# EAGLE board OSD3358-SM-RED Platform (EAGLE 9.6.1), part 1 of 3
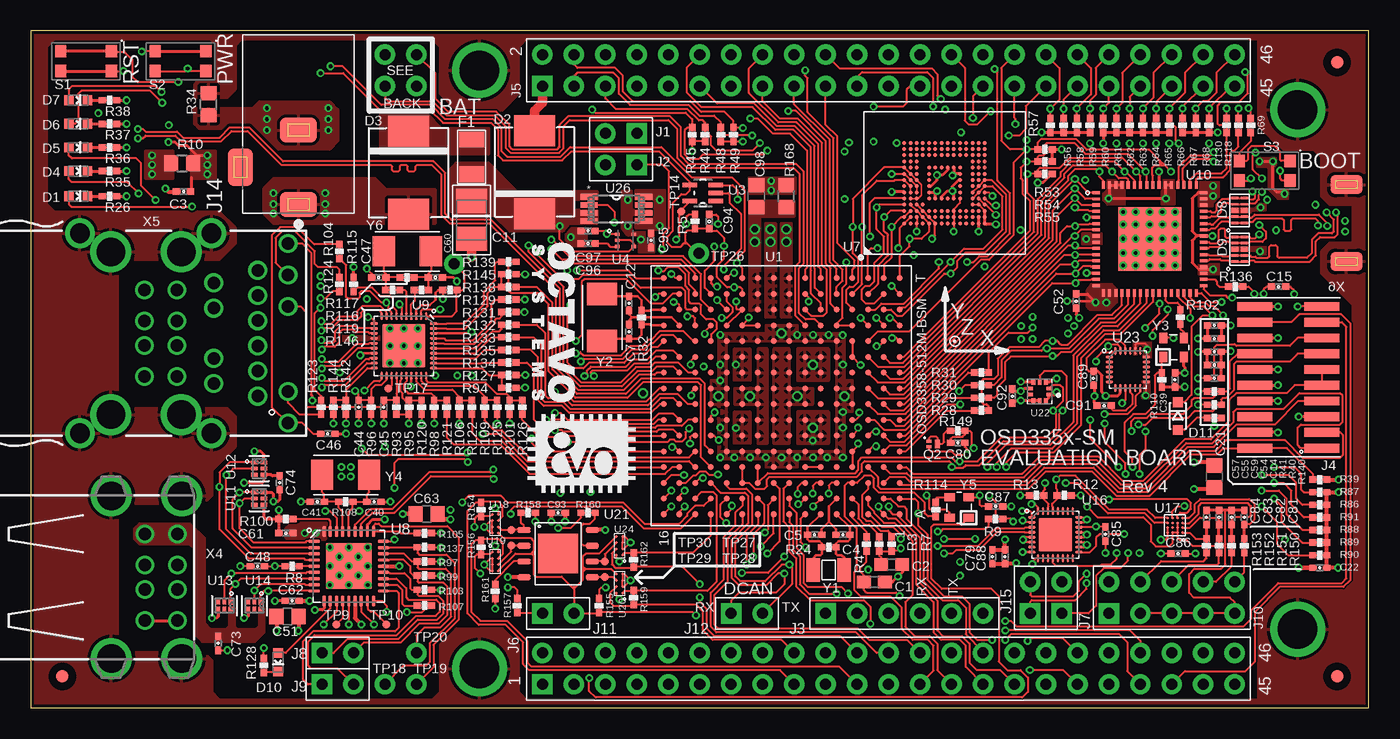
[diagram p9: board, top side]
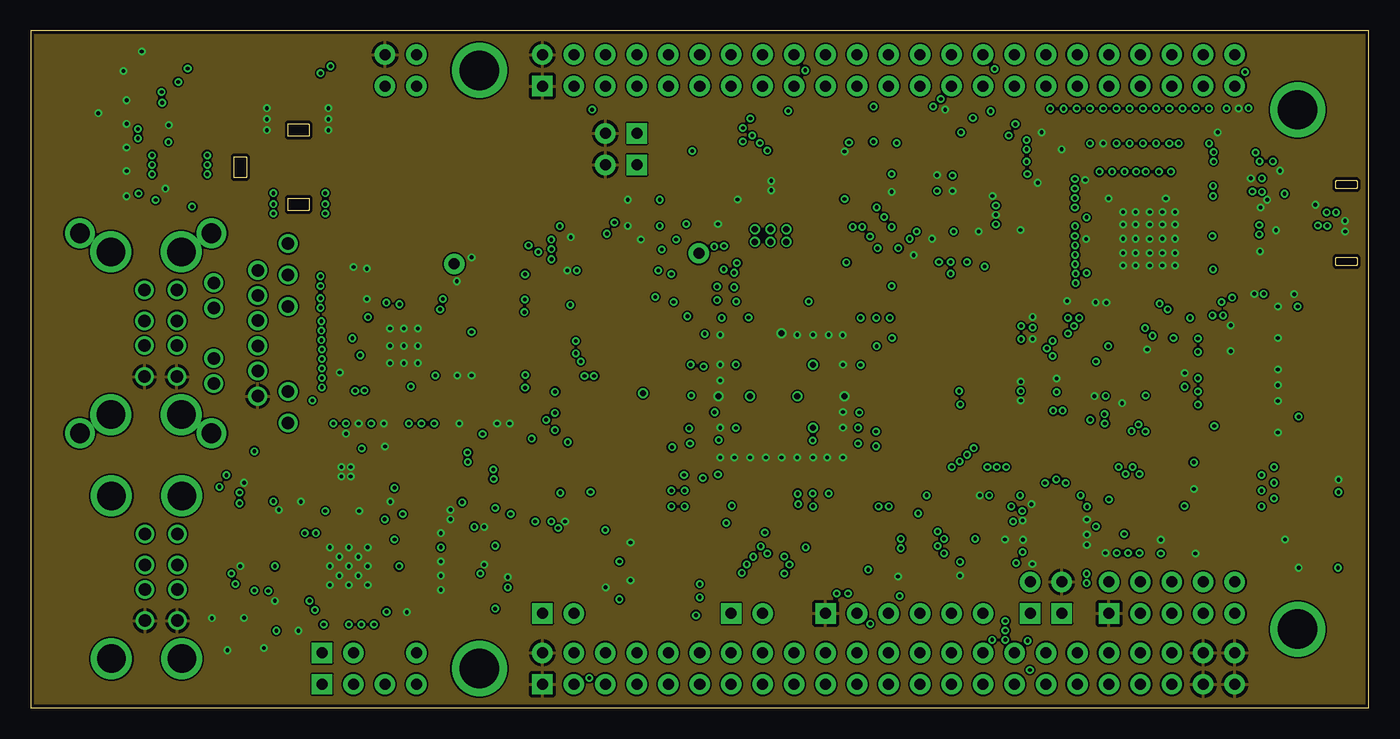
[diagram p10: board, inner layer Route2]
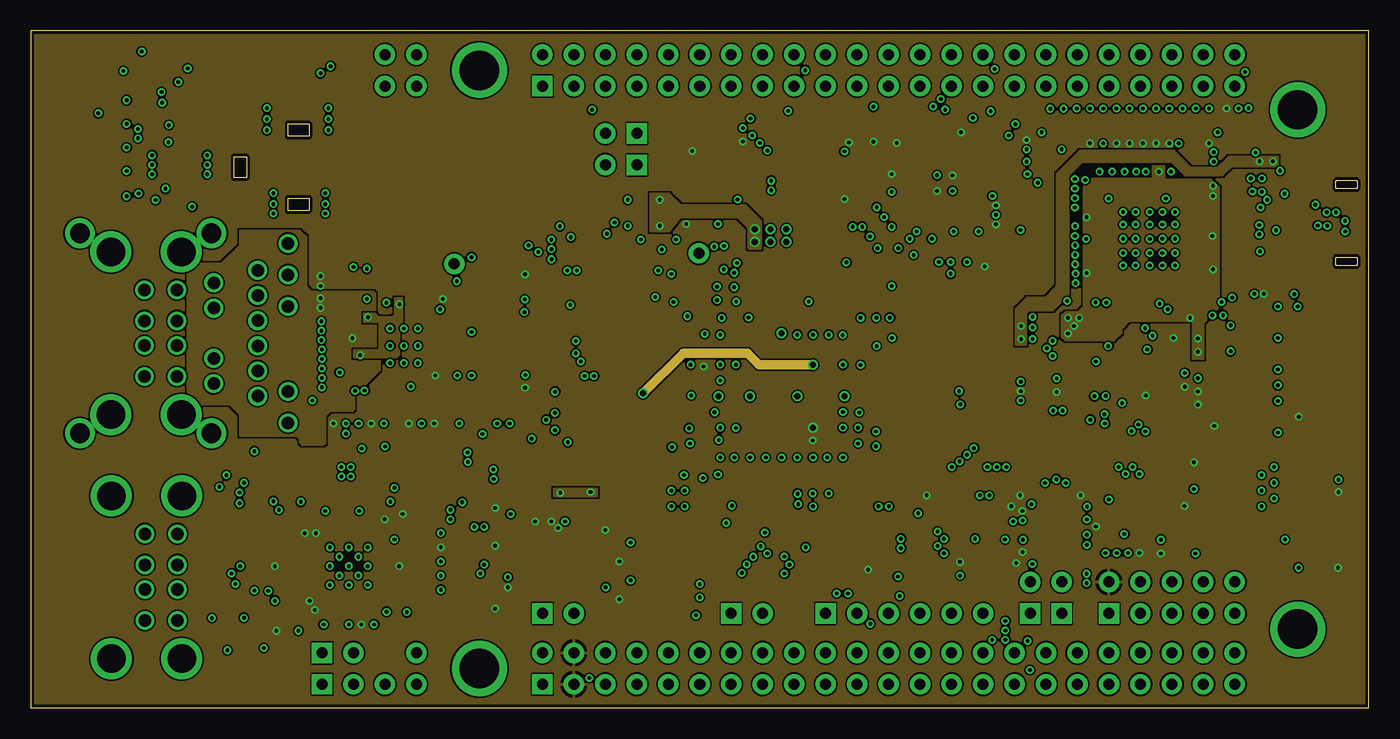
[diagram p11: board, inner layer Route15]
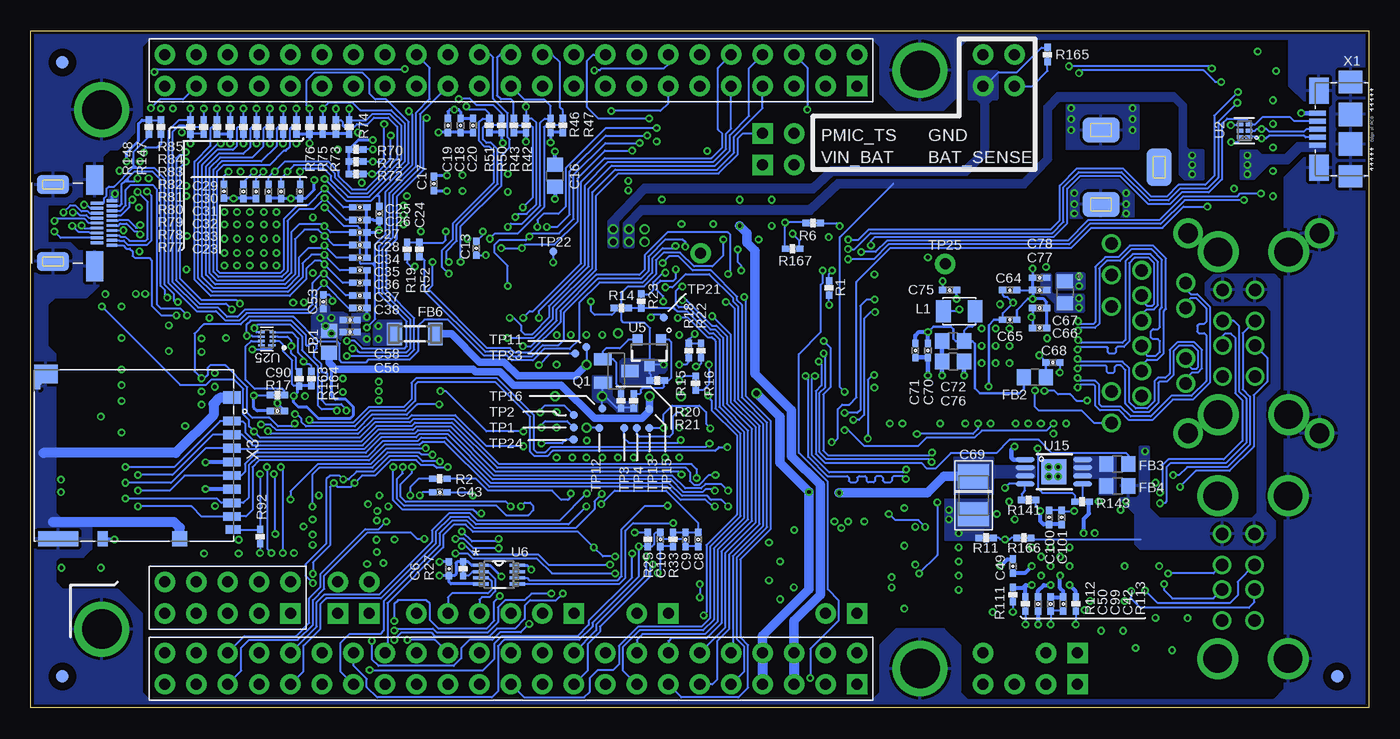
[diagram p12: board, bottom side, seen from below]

Size 107.95 x 54.61 mm. Coordinates in mm from the lower left corner, seen from the top.
Outline: 0,0 107.95,0 107.95,54.61 0,54.61 0,0
Copper layers (1*2*15*16): Top 0.035mm / dielectric 0.23mm / Route2 0.035mm / dielectric 0.93mm / Route15 0.035mm / dielectric 0.23mm / Bottom 0.035mm
Design rules "MF_Standard_4_Layer *": minimum track width 5mil, minimum drill 12mil, track to track 5mil, track to pad 5mil, pad to pad 5mil, via to via 5mil, smd to smd 0mil, copper to edge 10mil, drill to drill 10mil, minimum pad ring 6mil, minimum via ring 6mil, stop-mask expansion 2mil, vias tented up to drill 25mil, thermal gap 10mil
Net classes: 0 default: width 0.127 mm, drill 0.254 mm; 1 ground: width 0.152 mm, drill 0.254 mm, clearance 0.152 mm

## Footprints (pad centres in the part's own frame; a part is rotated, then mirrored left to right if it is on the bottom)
C0603 = smd 1.1 x 1: 1 -0.85,0; 2 0.85,0
C0402 = smd 0.61 x 0.508: 1 -0.559,0; 2 0.559,0
B/3528-21R = smd 1.95 x 2.5: + 1.525,0; - -1.525,0
C0805 = smd 1.143 x 1.27: 1 -0.889,0; 2 0.889,0
0603 = smd 0.787 x 0.787: 1 -0.749,0; 2 0.749,0
SMC = smd 2.5 x 3.3: A 3.35,0; C -3.35,0
10-USON(2.5X1) = smd 0.2 x 0.565: 1 -1,0.385; 2 -0.5,0.385; 4 0.5,0.385; 5 1,0.385; 6 1,-0.385; 7 0.5,-0.385; 9 -0.5,-0.385; 10 -1,-0.385 | smd 0.4 x 0.565: 3 0,0.385; 8 0,-0.385
SOD323(NXP)REFLOW = smd 0.8 x 0.8: A 1.125,0; C -1.125,0
F1206W = smd 1.27 x 2.032: 1 -1.397,0; 2 1.397,0
SM-1206 = smd 1.2 x 1.8: 1 -1.65,0; 2 1.65,0
FIDUCIAL_40MIL = smd 1.016 x 1.016: P$1 0,0
H2-2.54 = drill 0.889 pad 1.651 square: 1 0,1.27 | drill 0.889 pad 1.651: 2 0,-1.27
H6-2.54 = drill 0.889 pad 1.651 square: 1 0,6.35 | drill 0.889 pad 1.651: 2 0,3.81; 3 0,1.27; 4 0,-1.27; 5 0,-3.81; 6 0,-6.35
2ROWS_10PINS_1.27MM_PITCH_ROW_2.54MM_PITCH_PIN6_KEYED = smd 2.794 x 0.711: 1 -2.705,5.715; 2 2.705,5.715; 3 -2.705,4.445; 4 2.705,4.445; 5 -2.705,3.175; 6 2.705,3.175; 7 -2.705,1.905; 8 2.705,1.905; 9 -2.705,0.635; 10 2.705,0.635; 11 -2.705,-0.635; 12 2.705,-0.635; 13 -2.705,-1.905; 14 2.705,-1.905; 15 -2.705,-3.175; 16 2.705,-3.175; 17 -2.705,-4.445; 18 2.705,-4.445; 19 -2.705,-5.715; 20 2.705,-5.715
H2X23-2.54 = drill 0.889 pad 1.651 square: 1 -1.27,27.94 | drill 0.889 pad 1.651: 2 1.27,27.94; 3 -1.27,25.4; 4 1.27,25.4; 5 -1.27,22.86; 6 1.27,22.86; 7 -1.27,20.32; 8 1.27,20.32; 9 -1.27,17.78; 10 1.27,17.78; 11 -1.27,15.24; 12 1.27,15.24; 13 -1.27,12.7; 14 1.27,12.7; 15 -1.27,10.16; 16 1.27,10.16; 17 -1.27,7.62; 18 1.27,7.62; 19 -1.27,5.08; 20 1.27,5.08; 21 -1.27,2.54; 22 1.27,2.54; 23 -1.27,0; 24 1.27,0; 25 -1.27,-2.54; 26 1.27,-2.54; 27 -1.27,-5.08; 28 1.27,-5.08; 29 -1.27,-7.62; 30 1.27,-7.62; 31 -1.27,-10.16; 32 1.27,-10.16; 33 -1.27,-12.7; 34 1.27,-12.7; 35 -1.27,-15.24; 36 1.27,-15.24; 37 -1.27,-17.78; 38 1.27,-17.78; 39 -1.27,-20.32; 40 1.27,-20.32; 41 -1.27,-22.86; 42 1.27,-22.86; 43 -1.27,-25.4; 44 1.27,-25.4; 45 -1.27,-27.94; 46 1.27,-27.94
H2X5-2.54 = drill 0.889 pad 1.651 square: 1 -1.27,5.08 | drill 0.889 pad 1.651: 2 1.27,5.08; 3 -1.27,2.54; 4 1.27,2.54; 5 -1.27,0; 6 1.27,0; 7 -1.27,-2.54; 8 1.27,-2.54; 9 -1.27,-5.08; 10 1.27,-5.08
CUI_PJ-102BH-DIM-SMT-PAD = smd 2 x 3: 1 -6.5,0; 2 -0.5,0 | smd 2 x 3 bottom: 1_B -6.5,0; 2_B -0.5,0 | smd 3 x 2: 3 -3.5,4.7 | smd 3 x 2 bottom: 3_B -3.5,4.7
CVH252009 = smd 1.2 x 1.75: P$1 -1.275,0; P$2 1.275,0
MOUNTING_HOLE = drill 3.175 pad 4.445: P$1 0,0
SOT23-BEC = smd 1 x 1.4: B -0.95,-1.1; C 0,1.1; E 0.95,-1.1
X1-DFN1006-3 = smd 0.4 x 0.25: B -0.35,0.225; E -0.35,-0.225 | smd 0.4 x 0.7: C 0.35,0
R0402 = smd 0.61 x 0.508: 1 -0.559,0; 2 0.559,0
R0805 = smd 1.143 x 1.27: 1 -0.889,0; 2 0.889,0
SW4SMD_63X161LS = smd 0.9 x 1: 1 2.05,0.8; 2 2.05,-0.8; 3 -2.05,0.8; 4 -2.05,-0.8
TP_B0,65 = smd 0.635 x 0.635: TP 0,0
TESTPAD/W_HOLE_1X1 = drill 0.889 pad 1.651: P$1 0,0
OSD335X-BGA-256 = smd 0.5 x 0.5: A1 -9.525,-9.525; A2 -9.525,-8.255; A3 -9.525,-6.985; A4 -9.525,-5.715; A5 -9.525,-4.445; A6 -9.525,-3.175; A7 -9.525,-1.905; A8 -9.525,-0.635; A9 -9.525,0.635; A10 -9.525,1.905; A11 -9.525,3.175; A12 -9.525,4.445; A13 -9.525,5.715; A14 -9.525,6.985; A15 -9.525,8.255; A16 -9.525,9.525; B1 -8.255,-9.525; B2 -8.255,-8.255; B3 -8.255,-6.985; B4 -8.255,-5.715; B5 -8.255,-4.445; B6 -8.255,-3.175; B7 -8.255,-1.905; B8 -8.255,-0.635; B9 -8.255,0.635; B10 -8.255,1.905; B11 -8.255,3.175; B12 -8.255,4.445; B13 -8.255,5.715; B14 -8.255,6.985; B15 -8.255,8.255; B16 -8.255,9.525; C1 -6.985,-9.525; C2 -6.985,-8.255; C3 -6.985,-6.985; C4 -6.985,-5.715; C5 -6.985,-4.445; C6 -6.985,-3.175; C7 -6.985,-1.905; C8 -6.985,-0.635; C9 -6.985,0.635; C10 -6.985,1.905; C11 -6.985,3.175; C12 -6.985,4.445; C13 -6.985,5.715; C14 -6.985,6.985; C15 -6.985,8.255; C16 -6.985,9.525; D1 -5.715,-9.525; D2 -5.715,-8.255; D3 -5.715,-6.985; D4 -5.715,-5.715; D5 -5.715,-4.445; D6 -5.715,-3.175; D7 -5.715,-1.905; D8 -5.715,-0.635; D9 -5.715,0.635; D10 -5.715,1.905; D11 -5.715,3.175; D12 -5.715,4.445; D13 -5.715,5.715; D14 -5.715,6.985; D15 -5.715,8.255; D16 -5.715,9.525; E1 -4.445,-9.525; E2 -4.445,-8.255; E3 -4.445,-6.985; E4 -4.445,-5.715; E5 -4.445,-4.445; E6 -4.445,-3.175; E7 -4.445,-1.905; E8 -4.445,-0.635; E9 -4.445,0.635; E10 -4.445,1.905; E11 -4.445,3.175; E12 -4.445,4.445; E13 -4.445,5.715; E14 -4.445,6.985; E15 -4.445,8.255; E16 -4.445,9.525; F1 -3.175,-9.525; F2 -3.175,-8.255; F3 -3.175,-6.985; F4 -3.175,-5.715; F5 -3.175,-4.445; F6 -3.175,-3.175; F7 -3.175,-1.905; F8 -3.175,-0.635; F9 -3.175,0.635; F10 -3.175,1.905; F11 -3.175,3.175; F12 -3.175,4.445; F13 -3.175,5.715; F14 -3.175,6.985; F15 -3.175,8.255; F16 -3.175,9.525; G1 -1.905,-9.525; G2 -1.905,-8.255; G3 -1.905,-6.985; G4 -1.905,-5.715; G5 -1.905,-4.445; G6 -1.905,-3.175; G7 -1.905,-1.905; G8 -1.905,-0.635; G9 -1.905,0.635; G10 -1.905,1.905; G11 -1.905,3.175; G12 -1.905,4.445; G13 -1.905,5.715; G14 -1.905,6.985; G15 -1.905,8.255; G16 -1.905,9.525; H1 -0.635,-9.525; H2 -0.635,-8.255; H3 -0.635,-6.985; H4 -0.635,-5.715; H5 -0.635,-4.445; H6 -0.635,-3.175; H7 -0.635,-1.905; H8 -0.635,-0.635; H9 -0.635,0.635; H10 -0.635,1.905; H11 -0.635,3.175; H12 -0.635,4.445; H13 -0.635,5.715; H14 -0.635,6.985; H15 -0.635,8.255; H16 -0.635,9.525; J1 0.635,-9.525; J2 0.635,-8.255; J3 0.635,-6.985; J4 0.635,-5.715; J5 0.635,-4.445; J6 0.635,-3.175; J7 0.635,-1.905; J8 0.635,-0.635; J9 0.635,0.635; J10 0.635,1.905; J11 0.635,3.175; J12 0.635,4.445; J13 0.635,5.715; J14 0.635,6.985; J15 0.635,8.255; J16 0.635,9.525; K1 1.905,-9.525; K2 1.905,-8.255; K3 1.905,-6.985; K4 1.905,-5.715; K5 1.905,-4.445; K6 1.905,-3.175; K7 1.905,-1.905; K8 1.905,-0.635; K9 1.905,0.635; K10 1.905,1.905; K11 1.905,3.175; K12 1.905,4.445; K13 1.905,5.715; K14 1.905,6.985; K15 1.905,8.255; K16 1.905,9.525; L1 3.175,-9.525; L2 3.175,-8.255; L3 3.175,-6.985; L4 3.175,-5.715; L5 3.175,-4.445; L6 3.175,-3.175; L7 3.175,-1.905; L8 3.175,-0.635; L9 3.175,0.635; L10 3.175,1.905; L11 3.175,3.175; L12 3.175,4.445; L13 3.175,5.715; L14 3.175,6.985; L15 3.175,8.255; L16 3.175,9.525; M1 4.445,-9.525; M2 4.445,-8.255; M3 4.445,-6.985; M4 4.445,-5.715; M5 4.445,-4.445; M6 4.445,-3.175; M7 4.445,-1.905; M8 4.445,-0.635; M9 4.445,0.635; M10 4.445,1.905; M11 4.445,3.175; M12 4.445,4.445; M13 4.445,5.715; M14 4.445,6.985; M15 4.445,8.255; M16 4.445,9.525; N1 5.715,-9.525; N2 5.715,-8.255; N3 5.715,-6.985; N4 5.715,-5.715; N5 5.715,-4.445; N6 5.715,-3.175; N7 5.715,-1.905; N8 5.715,-0.635; N9 5.715,0.635; N10 5.715,1.905; N11 5.715,3.175; N12 5.715,4.445; N13 5.715,5.715; N14 5.715,6.985; N15 5.715,8.255; N16 5.715,9.525; P1 6.985,-9.525; P2 6.985,-8.255; P3 6.985,-6.985; P4 6.985,-5.715; P5 6.985,-4.445; P6 6.985,-3.175; P7 6.985,-1.905; P8 6.985,-0.635; P9 6.985,0.635; P10 6.985,1.905; P11 6.985,3.175; P12 6.985,4.445; P13 6.985,5.715; P14 6.985,6.985; P15 6.985,8.255; P16 6.985,9.525; R1 8.255,-9.525; R2 8.255,-8.255; R3 8.255,-6.985; R4 8.255,-5.715; R5 8.255,-4.445; R6 8.255,-3.175; R7 8.255,-1.905; R8 8.255,-0.635; R9 8.255,0.635; R10 8.255,1.905; R11 8.255,3.175; R12 8.255,4.445; R13 8.255,5.715; R14 8.255,6.985; R15 8.255,8.255; R16 8.255,9.525; T1 9.525,-9.525; T2 9.525,-8.255; T3 9.525,-6.985; T4 9.525,-5.715; T5 9.525,-4.445; T6 9.525,-3.175; T7 9.525,-1.905; T8 9.525,-0.635; T9 9.525,0.635; T10 9.525,1.905; T11 9.525,3.175; T12 9.525,4.445; T13 9.525,5.715; T14 9.525,6.985; T15 9.525,8.255; T16 9.525,9.525
6-SON(1.45X1) = smd 0.55 x 0.3: 1 -0.355,0.5 | smd 0.52 x 0.3: 2 -0.37,0; 3 -0.37,-0.5; 4 0.37,-0.5; 5 0.37,0; 6 0.37,0.5
SC-70-5 = smd 1.168 x 0.356: 1 -1.041,0.65; 2 -1.041,0; 3 -1.041,-0.65; 4 1.041,-0.65; 5 1.041,0.65
5-VSOF(1.6X1.6MM) = smd 0.35 x 0.25: 1 -0.675,0.5; 2 -0.675,0; 3 -0.675,-0.5; 4 0.675,-0.5; 5 0.675,0.5
SOT23-3 = smd 0.8 x 0.9: 1 -0.95,-1; 2 0.95,-1; 3 0,1.1
8-VSSOP(2.3X2MM) = smd 1.27 x 0.254: 1 -1.473,0.749; 2 -1.473,0.249; 3 -1.473,-0.249; 4 -1.473,-0.749; 5 1.473,-0.749; 6 1.473,-0.249; 7 1.473,0.249; 8 1.473,0.749
153-WFBGA(11X10) = smd 0.305 x 0.305: A1 -3.25,3.25; A2 -2.75,3.25; A3 -2.25,3.25; A4 -1.75,3.25; A5 -1.25,3.25; A6 -0.75,3.25; A7 -0.25,3.25; A8 0.25,3.25; A9 0.75,3.25; A10 1.25,3.25; A11 1.75,3.25; A12 2.25,3.25; A13 2.75,3.25; A14 3.25,3.25; B1 -3.25,2.75; B2 -2.75,2.75; B3 -2.25,2.75; B4 -1.75,2.75; B5 -1.25,2.75; B6 -0.75,2.75; B7 -0.25,2.75; B8 0.25,2.75; B9 0.75,2.75; B10 1.25,2.75; B11 1.75,2.75; B12 2.25,2.75; B13 2.75,2.75; B14 3.25,2.75; C1 -3.25,2.25; C2 -2.75,2.25; C3 -2.25,2.25; C4 -1.75,2.25; C5 -1.25,2.25; C6 -0.75,2.25; C7 -0.25,2.25; C8 0.25,2.25; C9 0.75,2.25; C10 1.25,2.25; C11 1.75,2.25; C12 2.25,2.25; C13 2.75,2.25; C14 3.25,2.25; D1 -3.25,1.75; D2 -2.75,1.75; D3 -2.25,1.75; D4 -1.75,1.75; D12 2.25,1.75; D13 2.75,1.75; D14 3.25,1.75; E1 -3.25,1.25; E2 -2.75,1.25; E3 -2.25,1.25; E5 -1.25,1.25; E6 -0.75,1.25; E7 -0.25,1.25; E8 0.25,1.25; E9 0.75,1.25; E10 1.25,1.25; E12 2.25,1.25; E13 2.75,1.25; E14 3.25,1.25; F1 -3.25,0.75; F2 -2.75,0.75; F3 -2.25,0.75; F5 -1.25,0.75; F10 1.25,0.75; F12 2.25,0.75; F13 2.75,0.75; F14 3.25,0.75; G1 -3.25,0.25; G2 -2.75,0.25; G3 -2.25,0.25; G5 -1.25,0.25; G10 1.25,0.25; G12 2.25,0.25; G13 2.75,0.25; G14 3.25,0.25; H1 -3.25,-0.25; H2 -2.75,-0.25; H3 -2.25,-0.25; H5 -1.25,-0.25; H10 1.25,-0.25; H12 2.25,-0.25; H13 2.75,-0.25; H14 3.25,-0.25; J1 -3.25,-0.75; J2 -2.75,-0.75; J3 -2.25,-0.75; J5 -1.25,-0.75; J10 1.25,-0.75; J12 2.25,-0.75; J13 2.75,-0.75; J14 3.25,-0.75; K1 -3.25,-1.25; K2 -2.75,-1.25; K3 -2.25,-1.25; K5 -1.25,-1.25; K6 -0.75,-1.25; K7 -0.25,-1.25; K8 0.25,-1.25; K9 0.75,-1.25; K10 1.25,-1.25; K12 2.25,-1.25; K13 2.75,-1.25; K14 3.25,-1.25; L1 -3.25,-1.75; L2 -2.75,-1.75; L3 -2.25,-1.75; L12 2.25,-1.75; L13 2.75,-1.75; L14 3.25,-1.75; M1 -3.25,-2.25; M2 -2.75,-2.25; M3 -2.25,-2.25; M4 -1.75,-2.25; M5 -1.25,-2.25; M6 -0.75,-2.25; M7 -0.25,-2.25; M8 0.25,-2.25; M9 0.75,-2.25; M10 1.25,-2.25; M11 1.75,-2.25; M12 2.25,-2.25; M13 2.75,-2.25; M14 3.25,-2.25; N1 -3.25,-2.75; N2 -2.75,-2.75; N3 -2.25,-2.75; N4 -1.75,-2.75; N5 -1.25,-2.75; N6 -0.75,-2.75; N7 -0.25,-2.75; N8 0.25,-2.75; N9 0.75,-2.75; N10 1.25,-2.75; N11 1.75,-2.75; N12 2.25,-2.75; N13 2.75,-2.75; N14 3.25,-2.75; P1 -3.25,-3.25; P2 -2.75,-3.25; P3 -2.25,-3.25; P4 -1.75,-3.25; P5 -1.25,-3.25; P6 -0.75,-3.25; P7 -0.25,-3.25; P8 0.25,-3.25; P9 0.75,-3.25; P10 1.25,-3.25; P11 1.75,-3.25; P12 2.25,-3.25; P13 2.75,-3.25; P14 3.25,-3.25
6-SQFN(6X6) = smd 0.9 x 0.28: 1 -2.8,2; 2 -2.8,1.5; 3 -2.8,1; 4 -2.8,0.5; 5 -2.8,0; 6 -2.8,-0.5; 7 -2.8,-1; 8 -2.8,-1.5; 9 -2.8,-2; 19 2.8,-2; 20 2.8,-1.5; 21 2.8,-1; 22 2.8,-0.5; 23 2.8,0; 24 2.8,0.5; 25 2.8,1; 26 2.8,1.5; 27 2.8,2 | smd 0.28 x 0.9: 10 -2,-2.8; 11 -1.5,-2.8; 12 -1,-2.8; 13 -0.5,-2.8; 14 0,-2.8; 15 0.5,-2.8; 16 1,-2.8; 17 1.5,-2.8; 18 2,-2.8; 28 2,2.8; 29 1.5,2.8; 30 1,2.8; 31 0.5,2.8; 32 0,2.8; 33 -0.5,2.8; 34 -1,2.8; 35 -1.5,2.8; 36 -2,2.8 | smd 3.7 x 3.7: 37 0,0
40-QFN(5X5MM) = smd 0.6 x 0.2: 1 -2.4,1.8; 2 -2.4,1.4; 3 -2.4,1; 4 -2.4,0.6; 5 -2.4,0.2; 6 -2.4,-0.2; 7 -2.4,-0.6; 8 -2.4,-1; 9 -2.4,-1.4; 10 -2.4,-1.8; 21 2.4,-1.8; 22 2.4,-1.4; 23 2.4,-1; 24 2.4,-0.6; 25 2.4,-0.2; 26 2.4,0.2; 27 2.4,0.6; 28 2.4,1; 29 2.4,1.4; 30 2.4,1.8 | smd 0.2 x 0.6: 11 -1.8,-2.4; 12 -1.4,-2.4; 13 -1,-2.4; 14 -0.6,-2.4; 15 -0.2,-2.4; 16 0.2,-2.4; 17 0.6,-2.4; 18 1,-2.4; 19 1.4,-2.4; 20 1.8,-2.4; 31 1.8,2.4; 32 1.4,2.4; 33 1,2.4; 34 0.6,2.4; 35 0.2,2.4; 36 -0.2,2.4; 37 -0.6,2.4; 38 -1,2.4; 39 -1.4,2.4; 40 -1.8,2.4 | smd 3.5 x 3.5: 41 0,0
64-HVQFN(9X9) = smd 0.6 x 0.25: 1 -4.35,3.75; 3 -4.35,2.75; 4 -4.35,2.25; 5 -4.35,1.75; 6 -4.35,1.25; 7 -4.35,0.75; 8 -4.35,0.25; 9 -4.35,-0.25; 10 -4.35,-0.75; 11 -4.35,-1.25; 12 -4.35,-1.75; 13 -4.35,-2.25; 14 -4.35,-2.75; 15 -4.35,-3.25; 16 -4.35,-3.75; 33 4.35,-3.75; 34 4.35,-3.25; 35 4.35,-2.75; 36 4.35,-2.25; 37 4.35,-1.75; 38 4.35,-1.25; 39 4.35,-0.75; 40 4.35,-0.25; 41 4.35,0.25; 42 4.35,0.75; 43 4.35,1.25; 44 4.35,1.75; 45 4.35,2.25; 46 4.35,2.75; 47 4.35,3.25; 48 4.35,3.75 | smd 0.6 x 0.2: 2 -4.35,3.25 | smd 0.25 x 0.6: 17 -3.75,-4.35; 18 -3.25,-4.35; 19 -2.75,-4.35; 20 -2.25,-4.35; 21 -1.75,-4.35; 22 -1.25,-4.35; 23 -0.75,-4.35; 24 -0.25,-4.35; 25 0.25,-4.35; 26 0.75,-4.35; 27 1.25,-4.35; 28 1.75,-4.35; 29 2.25,-4.35; 30 2.75,-4.35; 31 3.25,-4.35; 32 3.75,-4.35; 49 3.75,4.35; 50 3.25,4.35; 51 2.75,4.35; 52 2.25,4.35; 53 1.75,4.35; 54 1.25,4.35; 55 0.75,4.35; 56 0.25,4.35; 57 -0.25,4.35; 58 -0.75,4.35; 59 -1.25,4.35; 60 -1.75,4.35; 61 -2.25,4.35; 62 -2.75,4.35; 63 -3.25,4.35; 64 -3.75,4.35 | smd 5.1 x 5.1: 65 0,0
8-TSSOP(3.00MM_WIDTH) = smd 1.524 x 0.406: 1 -2.311,0.975; 2 -2.324,0.325; 3 -2.324,-0.325; 4 -2.324,-0.975; 5 2.324,-0.975; 6 2.324,-0.325; 7 2.324,0.325; 8 2.311,0.975 | smd 2.032 x 2.032: TH 0,0
QFN32-0.4-4X4MM = smd 0.6 x 0.2: 1 -1.9,1.4; 2 -1.9,1; 3 -1.9,0.6; 4 -1.9,0.2; 5 -1.9,-0.2; 6 -1.9,-0.6; 7 -1.9,-1; 8 -1.9,-1.4; 17 1.9,-1.4; 18 1.9,-1; 19 1.9,-0.6; 20 1.9,-0.2; 21 1.9,0.2; 22 1.9,0.6; 23 1.9,1; 24 1.9,1.4 | smd 0.2 x 0.6: 9 -1.4,-1.9; 10 -1,-1.9; 11 -0.6,-1.9; 12 -0.2,-1.9; 13 0.2,-1.9; 14 0.6,-1.9; 15 1,-1.9; 16 1.4,-1.9; 25 1.4,1.9; 26 1,1.9; 27 0.6,1.9; 28 0.2,1.9; 29 -0.2,1.9; 30 -0.6,1.9; 31 -1,1.9; 32 -1.4,1.9 | smd 2.7 x 2.7: 33 0,0
16-DSBGA = smd 0.23 x 0.23: A1 -0.6,-0.6; A2 -0.6,-0.2; A3 -0.6,0.2; A4 -0.6,0.6; B1 -0.2,-0.6; B2 -0.2,-0.2; B3 -0.2,0.2; B4 -0.2,0.6; C1 0.2,-0.6; C2 0.2,-0.2; C3 0.2,0.2; C4 0.2,0.6; D1 0.6,-0.6; D2 0.6,-0.2; D3 0.6,0.2; D4 0.6,0.6
8-DSBGA(1.9X0.9) = smd 0.23 x 0.23: A1 -0.25,0.75; A2 0.25,0.75; B1 -0.25,0.25; B2 0.25,0.25; C1 -0.25,-0.25; C2 0.25,-0.25; D1 -0.25,-0.75; D2 0.25,-0.75
8-WSON(5X6MM) = smd 1.05 x 0.45: 1 -2.75,1.905; 2 -2.75,0.635; 3 -2.75,-0.635; 4 -2.75,-1.905; 5 2.75,-1.905; 6 2.75,-0.635; 7 2.75,0.635; 8 2.75,1.905 | smd 3.2 x 3.2: PAD 0,0
10-HLGA(2X2MM) = smd 0.387 x 0.3: 1 -0.745,0.25; 2 -0.745,-0.25; 6 0.745,-0.25; 7 0.745,0.25 | smd 0.3 x 0.387: 3 -0.5,-0.745; 4 0,-0.745; 5 0.5,-0.745; 8 0.5,0.745; 9 0,0.745; 10 -0.5,0.745
24-QFN(3X3) = smd 0.6 x 0.2: 1 -1.5,1; 2 -1.5,0.6; 3 -1.5,0.2; 4 -1.5,-0.2; 5 -1.5,-0.6; 6 -1.5,-1; 13 1.5,-1; 14 1.5,-0.6; 15 1.5,-0.2; 16 1.5,0.2; 17 1.5,0.6; 18 1.5,1 | smd 0.2 x 0.6: 7 -1,-1.5; 8 -0.6,-1.5; 9 -0.2,-1.5; 10 0.2,-1.5; 11 0.6,-1.5; 12 1,-1.5; 19 1,1.5; 20 0.6,1.5; 21 0.2,1.5; 22 -0.2,1.5; 23 -0.6,1.5; 24 -1,1.5
8-X2SON(1.4X1.0) = smd 0.6 x 0.175: 1 -0.4,0.525 | smd 0.5 x 0.175: 2 -0.45,0.175; 3 -0.45,-0.175; 4 -0.45,-0.525; 5 0.45,-0.525; 6 0.45,-0.175; 7 0.45,0.175; 8 0.45,0.525
8-VSSOP(3X3MM) = smd 1.4 x 0.45: 1 -2.2,0.975; 2 -2.2,0.325; 3 -2.2,-0.325; 4 -2.2,-0.975; 5 2.2,-0.975; 6 2.2,-0.325; 7 2.2,0.325; 8 2.2,0.975
MICRO_USB_2.0_RECEP_5POS_SMD_RIGHT_ANGLE = smd 1.8 x 1.9: CGND1 -3.8,0; CGND4 3.8,0 | smd 1.9 x 1.9: CGND2 -1.2,0; CGND3 1.2,0 | smd 2.1 x 1.6: CGND5 3.1,2.55; CGND6 -3.1,2.55 | smd 0.4 x 1.35: D+ 0,2.675; D- -0.65,2.675; GND 1.3,2.675; ID 0.65,2.675; VBUS -1.3,2.675
10(8+2)POS_MICRO_SD_SMD_RIGHT_ANGLE = smd 0.7 x 1.4: 1 -3.2,15.95; 2 -2.1,15.95; 3 -1,15.95; 4 0.1,15.95; 5 1.2,15.95; 6 2.3,15.95; 7 3.4,15.95; 8 4.5,15.95 | smd 0.7 x 1.2: CD 5.55,16.05 | smd 0.5 x 0.5: CGND1 -6,0.25 | smd 1.5 x 1.9: CGND2 -7,0.95 | smd 0.21 x 0.21 rotated 45: CGND3 -6.25,0.5 | smd 1 x 1.4: CGND4 -5.1,15.95 | smd 1.2 x 1.2: CGND5 6.3,11.75 | smd 1.2 x 3.2: CGND6 6.3,1.95 | smd 1.2 x 0.8: GND 6.3,5.55
USB_HOST_HORIZONTAL_W/CHASSIS_GND_DUAL = drill 1: 1 -3.5,13.01; 2 -1,13.01; 3 1,13.01; 4 3.5,13.01; 5 -3.5,15.63; 6 -1,15.63; 7 1,15.63; 8 3.5,15.63 | drill 2.3: 9 -6.57,10.3; 10 6.57,10.3; 11 -6.57,15.98; 12 6.57,15.98
RJ45_10/100/1000_DUAL_USB_A_THRUHOLE_CONN = drill 1.016 pad 1.524: 1 5.075,22.11; 2 3.045,22.11; 3 1.015,22.11; 4 -1.015,22.11; 5 -3.045,22.11; 6 -5.075,22.11; 7 4.06,18.56; 8 2.03,18.56; 9 -2.03,18.56; 10 -4.06,18.56; 11 7.24,24.55; 12 4.7,24.55; 13 -2.16,24.55; 14 -4.7,24.55; 15 -7.24,24.55 | drill 1.6 pad 2.286: S1 -8.07,7.76; S2 8.07,7.76; S3 -8.07,18.38; S4 8.07,18.38 | drill 2.3 pad 3: S5 -6.57,10.26; S6 6.57,10.26; S7 -6.57,15.94; S8 6.57,15.94 | drill 1: U11 -3.5,12.97; U12 -1,12.97; U13 1,12.97; U14 3.5,12.97; U21 -3.5,15.59; U22 -1,15.59; U23 1,15.59; U24 3.5,15.59
MICRO_HDMI_19POS_SMD&THRUHOLE_RIGHT_ANGLE = smd 0.23 x 1: 1 1.6,3.54; 2 1.2,3.54; 3 0.8,3.54; 4 0.4,3.54; 5 0,3.54; 6 -0.4,3.54; 7 -0.8,3.54; 8 -1.2,3.54; 9 -1.6,3.54 | smd 0.23 x 0.85: 10 -1.8,4.775; 11 -1.4,4.775; 12 -1,4.775; 13 -0.6,4.775; 14 -0.2,4.775; 15 0.2,4.775; 16 0.6,4.775; 17 1,4.775; 18 1.4,4.775; 19 1.8,4.775 | smd 2.4 x 1.38: 20 -3.48,3.37; 21 3.48,3.37 | smd 1.55 x 2.6: 22 -3.1,0; 23 3.1,0 | smd 1.55 x 2.6 bottom: 22_B -3.1,0; 23_B 3.1,0
2-SMD,NO_LEAD(3.2X1.5MM) = smd 1.1 x 1.9: P$1 -1.25,0; P$2 1.25,0
2-SMD,NO_LEAD(5X3.2MM) = smd 1.788 x 2.413: P$1 1.9,0; P$2 -1.9,0
4-SMD,NO_LEAD(2.5X2MM) = smd 0.65 x 0.85: 1 -0.825,-0.775; 2 0.825,-0.775; 3 0.825,0.775; 4 -0.825,0.775

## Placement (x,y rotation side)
C1  DNI  [C0603]  68.07,10.16 180 top
C2  DNI  [C0603]  69.47,11.56 180 top
C3  0.1uF  [C0402]  12.32,41.66 180 top
C4  18pF  [C0402]  65.53,13.97 180 top
C5  18pF  [C0402]  63.25,13.97 0 top
C6  0.1uF  [C0402]  74.22,11.23 90 bottom
C7  18pF  [C0402]  48.26,30.35 90 top
C8  1nF  [C0402]  54.1,13.59 270 bottom
C9  0.1uF  [C0402]  55.12,13.59 270 bottom
C10  0.1uF  [C0402]  57.15,13.59 90 bottom
C11  220uF  [B/3528-21R]  35.56,39.37 90 top
C12  18pF  [C0402]  48.26,32.64 270 top
C13  2.2uF  [C0402]  72.01,37.08 90 bottom
C14  0.1uF  [C0402]  95.5,26.59 0 top
C15  0.1uF  [C0402]  100.69,33.99 0 top
C16  10uF  [C0805]  65.66,42.93 270 bottom
C17  0.1uF  [C0402]  75.44,42.29 90 bottom
C18  0.1uF  [C0402]  73.28,46.99 270 bottom
C19  0.1uF  [C0402]  74.3,46.99 270 bottom
C20  0.1uF  [C0402]  72.26,46.99 270 bottom
C21  10uF  [C0805]  95.5,18.67 270 top
C22  0.1uF  [C0402]  104.01,11.3 180 top
C23  47pF  [C0402]  86.23,41.66 270 bottom
C24  47pF  [C0402]  79.83,39.88 270 bottom
C25  47pF  [C0402]  81.41,40.39 0 bottom
C26  47pF  [C0402]  81.41,39.37 0 bottom
C27  47pF  [C0402]  81.41,38.35 0 bottom
C28  47pF  [C0402]  81.41,37.34 0 bottom
C29  47pF  [C0402]  92.38,41.68 270 bottom
C30  47pF  [C0402]  90.81,41.66 270 bottom
C31  47pF  [C0402]  89.79,41.66 270 bottom
C32  47pF  [C0402]  88.77,41.66 270 bottom
C33  47pF  [C0402]  87.76,41.66 270 bottom
C34  47pF  [C0402]  81.41,36.32 0 bottom
C35  47pF  [C0402]  81.41,35.31 0 bottom
C36  47pF  [C0402]  81.41,34.29 0 bottom
C37  47pF  [C0402]  81.41,33.27 0 bottom
C38  47pF  [C0402]  81.41,32.26 0 bottom
C39  0.1uF  [C0402]  92.33,26.47 90 top
C40  18pF  [C0402]  27.69,16.64 0 top
C41  18pF  [C0402]  23.11,16.64 180 top
C42  1uF  [C0402]  24.64,8.38 90 bottom
C43  0.1uF  [C0402]  74.96,17.4 180 bottom
C44  470pF  [C0402]  26.44,24.26 270 top
C45  470pF  [C0402]  28.47,24.26 270 top
C46  470pF  [C0402]  23.95,22.12 0 top
C47  30pF  [C0402]  28.07,34.72 180 top
C48  0.1uF  [C0402]  18.29,11.43 180 top
C49  0.1uF  [C0402]  28.7,11.43 270 bottom
C50  0.1uF  [C0402]  26.67,8.38 90 bottom
C51  10uF  [C0805]  20.7,7.37 0 top
C52  2.2uF  [C0402]  84.35,32.82 90 top
C53  0.1uF  [C0402]  84.35,32.77 90 bottom
C54  2.2uF  [C0402]  95.5,27.66 0 top
C55  0.1uF  [C0402]  95.5,29.79 0 top
C56  2.2uF  [C0402]  82.19,30.33 0 bottom
C57  0.1uF  [C0402]  95.5,30.86 0 top
C58  0.1uF  [C0402]  82.19,31.29 0 bottom
C59  2.2uF  [C0402]  95.5,28.73 0 top
C60  30pF  [C0402]  32.64,34.72 0 top
C61  0.1uF  [C0402]  20.57,14.1 180 top
C62  0.1uF  [C0402]  21.08,8.64 180 top
C63  10uF  [C0805]  31.93,15.65 0 top
C64  0.1uF  [C0402]  28.96,33.71 0 bottom
C65  1uF  [C0402]  28.96,31.31 0 bottom
C66  0.1uF  [C0402]  26.54,30.66 0 bottom
C67  0.1uF  [C0402]  26.54,32.26 0 bottom
C68  0.1uF  [C0402]  25.48,27.86 0 bottom
C69  220uF  [B/3528-21R]  31.88,17.14 90 bottom
C70  0.1uF  [C0402]  35.56,28.83 270 bottom
C71  0.1uF  [C0402]  36.58,28.83 270 bottom
C72  10uF  [C0805]  33.53,29.59 180 bottom
C73  0.1uF  [C0402]  15.11,5.21 270 top
C74  0.1uF  [C0402]  20.07,18.16 90 top
C75  0.1uF  [C0402]  33.81,33.71 180 bottom
C76  10uF  [C0805]  33.53,27.94 180 bottom
C77  0.1uF  [C0402]  26.54,33.71 180 bottom
C78  1uF  [C0402]  26.54,34.7 180 bottom
C79  0.1uF  [C0402]  77.6,12.19 90 top
C80  1nF  [C0402]  74.8,21.39 0 top
C81  1nF  [C0402]  97.92,15.37 90 top
C82  1nF  [C0402]  96.9,15.37 90 top
C83  1nF  [C0402]  95.89,15.37 90 top
C84  1nF  [C0402]  94.87,15.37 90 top
C85  2200pF  [C0402]  86.72,14.02 270 top
C86  0.1uF  [C0402]  92.58,12.45 0 top
C87  2200pF  [C0402]  77.85,16.26 180 top
C88  2200pF  [C0402]  78.61,12.19 90 top
C89  0.1uF  [C0402]  85.75,26.59 270 top
C90  0.1uF  [C0402]  88.06,23.95 180 bottom
C91  0.1uF  [C0402]  86.61,24.38 180 top
C92  0.1uF  [C0402]  79.2,25.15 270 top
C93  0.1uF  [C0402]  42.55,15.75 0 top
C94  2.2uF  [C0402]  54.74,39.24 90 top
C95  0.1uF  [C0402]  50.04,37.72 270 top
C96  0.15uF  [C0402]  44.96,37.47 180 top
C97  1nF  [C0402]  44.96,38.48 180 top
C98  DNP  [C0805]  58.55,41.27 90 top
C99  0.1uF  [C0402]  25.65,8.38 90 bottom
C100  0.1uF, DNP  [C0402]  25.78,15.37 270 bottom
C101  1uF, DNP  [C0402]  24.77,15.37 270 bottom
D1  LTST-C191TBKT  [0603]  3.81,41.27 0 top
D2  SMCJ15CA  [SMC]  40.64,43.23 90 top
D3  B520C-13-F  [SMC]  30.48,43.18 270 top
D4  LTST-C191TBKT  [0603]  3.81,43.31 0 top
D5  LTST-C191TBKT  [0603]  3.81,45.21 0 top
D6  LTST-C191TBKT  [0603]  3.81,47.12 0 top
D7  LTST-C191TBKT  [0603]  3.81,49.02 0 top
D8  TPD4E05U06-Q1  [10-USON(2.5X1)]  97.54,40.13 90 top
D9  TPD4E05U06-Q1  [10-USON(2.5X1)]  97.54,37.01 90 top
D10  LTST-C191TBKT  [0603]  19.94,3.68 270 top
D11  RB751V40,115  [SOD323(NXP)REFLOW]  92.56,23.55 270 top
F1  4A Fuse  [F1206W]  35.56,44.45 270 top
FB1  150ohm, 800mA  [C0805]  83.9,29.54 270 bottom
FB2  150ohm, 800mA  [C0805]  26.92,26.67 180 bottom
FB3  600ohm, 0805  [C0805]  20.27,19.68 180 bottom
FB4  150ohm, 800mA  [C0805]  20.27,17.91 0 bottom
FB5  150ohm, 800mA  [C0805]  24.5,33.54 270 bottom
FB6  1206L025YR  [SM-1206]  76.96,30.18 180 bottom
FUD1  FIDUCIAL  [FIDUCIAL_40MIL]  105.41,2.54 0 top
FUD2  FIDUCIAL  [FIDUCIAL_40MIL]  105.41,52.07 0 top
FUD3  FIDUCIAL  [FIDUCIAL_40MIL]  2.54,2.54 0 top
FUD4  FIDUCIAL  [FIDUCIAL_40MIL]  105.41,52.07 90 bottom
FUD5  FIDUCIAL  [FIDUCIAL_40MIL]  2.54,2.54 90 bottom
FUD6  FIDUCIAL  [FIDUCIAL_40MIL]  105.41,2.54 90 bottom
J1  [H2-2.54]  47.62,46.35 270 top
J2  [H2-2.54]  47.62,43.81 270 top
J3  6p-2.54  [H6-2.54]  70.48,7.62 90 top
J4  FTR-110-51-L-D-06  [2ROWS_10PINS_1.27MM_PITCH_ROW_2.54MM_PITCH_PIN6_KEYED]  101.47,26.67 180 top
J5  S2012EC-23-ND  [H2X23-2.54]  69.22,51.44 90 top
J6  S2012EC-23-ND  [H2X23-2.54]  69.22,3.17 90 top
J7  [H2-2.54]  83.19,8.89 180 top
J8  [H2-2.54]  24.77,4.45 90 top
J9  [H2-2.54]  24.77,1.91 90 top
J10  TH-2X5  [H2X5-2.54]  92.08,8.89 90 top
J11  [H2-2.54]  42.55,7.62 90 top
J12  [H2-2.54]  57.78,7.62 90 top
J14  PJ-102BH-PAD  [CUI_PJ-102BH-DIM-SMT-PAD]  21.59,47.12 90 top
J15  [H2-2.54]  80.64,8.89 180 top
L1  CVH252009-4R7M  [CVH252009]  33.02,32 0 bottom
MGT1  MOUNTING_HOLE  [MOUNTING_HOLE]  36.2,3.17 0 top
MGT2  MOUNTING_HOLE  [MOUNTING_HOLE]  102.23,6.35 0 top
MGT3  MOUNTING_HOLE  [MOUNTING_HOLE]  36.2,51.44 0 top
MGT4  MOUNTING_HOLE  [MOUNTING_HOLE]  102.23,48.26 0 top
Q1  MMBT2907  [SOT23-BEC]  60.71,27.18 270 bottom
Q2  MMBT3904LP-7B  [X1-DFN1006-3]  72.82,21.29 0 top
R1  10K  [R0402]  43.54,33.88 90 bottom
R2  0  [R0402]  74.96,18.49 180 bottom
R3  0  [R0402]  68.45,13.21 270 top
R4  0  [R0402]  67.44,13.21 270 top
R5  10K  [R0402]  53.59,39.24 270 top
R6  10K  [R0402]  44.83,39.12 0 bottom
R7  0  [R0402]  69.47,13.21 270 top
R8  0, DNP  [R0402]  21.08,11.43 180 top
R9  0  [R0402]  77.85,15.24 0 top
R10  0, 1/8W  [R0805]  12.19,43.94 0 top
R11  100K  [R0402]  30.86,13.72 180 bottom
R12  1.5K  [R0402]  83.39,17.14 0 top
R13  1.5K  [R0402]  81.15,17.14 180 top
R14  0  [R0402]  60.3,32.26 0 bottom
R15  40.2K  [R0402]  57.4,26.42 0 bottom
R16  0  [R0402]  54.31,26.19 270 bottom
R17  200K  [R0402]  88.06,25.25 180 bottom
R18  4.75K  [R0402]  54.86,28.83 90 bottom
R19  0  [R0402]  76.61,36.98 90 bottom
R20  10.0K  [R0402]  59.31,24.77 270 bottom
R21  499  [R0402]  60.33,24.77 270 bottom
R22  4.75K  [R0402]  53.87,28.83 270 bottom
R23  0  [R0402]  58.7,32.82 270 bottom
R24  1M, DNI  [R0402]  64.39,12.95 180 top
R25  0  [R0402]  58.17,13.59 270 bottom
R26  1.5K  [R0402]  6.34,41.27 0 top
R27  100K  [R0402]  73.08,11.23 270 bottom
R28  0  [R0402]  76.71,24 0 top
R29  0  [R0402]  76.71,25.02 0 top
R30  0  [R0402]  76.71,26.04 0 top
R31  22  [R0402]  76.71,27.05 0 top
R32  1M  [R0402]  49.28,31.5 90 top
R33  0  [R0402]  56.13,13.59 270 bottom
R34  .1, 1/8W  [R0805]  14.35,48.69 90 top
R35  1.5K  [R0402]  6.35,43.31 0 top
R36  1.5K  [R0402]  6.35,45.21 0 top
R37  1.5K  [R0402]  6.35,47.12 0 top
R38  1.5K  [R0402]  6.35,49.02 0 top
R39  4.75K  [R0402]  104.01,18.41 180 top
R40  4.75K  [R0402]  95.5,24.46 180 top
R41  4.75K  [R0402]  95.5,25.53 180 top
R42  10K  [R0402]  68,46.99 270 bottom
R43  10K  [R0402]  68.99,46.99 270 bottom
R44  10K  [R0402]  54.41,46.25 270 top
R45  10K  [R0402]  53.37,46.25 270 top
R46  10K  [R0402]  66.01,46.99 270 bottom
R47  10K  [R0402]  65.02,46.99 270 bottom
R48  10K  [R0402]  55.68,46.25 270 top
R49  10K  [R0402]  56.69,46.25 270 top
R50  10K  [R0402]  69.98,46.99 270 bottom
R51  10K  [R0402]  70.97,46.99 270 bottom
R52  10K  [R0402]  77.6,36.98 270 bottom
R53  100K  [R0402]  81.84,45.06 180 top
R54  100K, DNI  [R0402]  81.84,44.07 180 top
R55  100K  [R0402]  81.84,43.08 180 top
R56  100K  [R0402]  83.34,46.99 90 top
R57  100K  [R0402]  82.27,46.99 90 top
R58  100K  [R0402]  84.4,46.99 90 top
R59  100K  [R0402]  85.47,46.99 90 top
R60  100K  [R0402]  86.54,46.99 90 top
R61  100K  [R0402]  87.6,46.99 90 top
R62  100K  [R0402]  88.67,46.99 90 top
R63  100K  [R0402]  89.74,46.99 90 top
R64  100K, DNI  [R0402]  90.81,46.99 90 top
R65  100K, DNI  [R0402]  91.87,46.99 90 top
R66  100K, DNI  [R0402]  92.94,46.99 90 top
R67  100K  [R0402]  94.01,46.99 90 top
R68  100K  [R0402]  95.07,46.99 90 top
R69  100  [R0402]  98.44,46.99 270 top
R70  100K, DNI  [R0402]  81.71,45.06 180 bottom
R71  100K  [R0402]  81.71,44.07 180 bottom
R72  100K, DNI  [R0402]  81.71,43.08 180 bottom
R73  100K, DNI  [R0402]  83.34,46.86 270 bottom
R74  100K, DNI  [R0402]  82.27,46.86 270 bottom
R75  100K, DNI  [R0402]  84.4,46.86 270 bottom
R76  100K, DNI  [R0402]  85.47,46.86 270 bottom
R77  100K, DNI  [R0402]  86.54,46.86 270 bottom
R78  100K, DNI  [R0402]  87.6,46.86 270 bottom
R79  100K, DNI  [R0402]  88.67,46.86 270 bottom
R80  100K, DNI  [R0402]  89.74,46.86 270 bottom
R81  100K  [R0402]  90.81,46.86 270 bottom
R82  100K  [R0402]  91.87,46.86 270 bottom
R83  100K  [R0402]  92.94,46.86 270 bottom
R84  100K, DNI  [R0402]  94.01,46.86 270 bottom
R85  100K, DNI  [R0402]  95.07,46.86 270 bottom
R86  10K  [R0402]  104.01,17.4 0 top
R87  10K  [R0402]  104.01,15.37 0 top
R88  10K  [R0402]  104.01,14.35 0 top
R89  10K  [R0402]  104.01,13.34 0 top
R90  10K  [R0402]  104.01,12.32 0 top
R91  10K  [R0402]  104.01,16.38 0 top
R92  10K  [R0402]  89.46,13.82 270 bottom
R93  10K  [R0402]  29.49,24.26 270 top
R94  10K  [R0402]  38.56,25.83 0 top
R95  10K  [R0402]  30.51,24.26 270 top
R96  10K  [R0402]  27.46,24.26 90 top
R97  100K  [R0402]  31.75,11.81 180 top
R98  10K  [R0402]  32.54,24.26 270 top
R99  100K  [R0402]  31.75,10.67 180 top
R100  12.0K  [R0402]  20.57,15.24 180 top
R101  10K  [R0402]  38.63,24.26 270 top
R102  22  [R0402]  92.76,31.52 90 top
R103  100K  [R0402]  31.75,9.53 180 top
R104  10K  [R0402]  24.89,36.83 90 top
R105  100K  [R0402]  31.75,14.1 180 top
R106  10K  [R0402]  34.57,24.26 90 top
R107  100K  [R0402]  31.75,8.26 180 top
R108  1M  [R0402]  25.4,16.64 180 top
R109  10K  [R0402]  37.62,24.26 90 top
R110  100K  [R0402]  91.26,26.47 270 top
R111  100K  [R0402]  28.7,9.14 270 bottom
R112  100K  [R0402]  27.69,8.38 270 bottom
R113  100K  [R0402]  23.62,8.38 270 bottom
R114  22  [R0402]  73.03,16 270 top
R115  2.37K  [R0402]  26.04,34.16 90 top
R116  22  [R0402]  29.18,33.71 180 top
R117  1M, DNI  [R0402]  30.35,34.72 180 top
R118  0  [R0402]  97.46,46.99 270 top
R119  0  [R0402]  31.52,33.71 0 top
R120  22  [R0402]  31.52,24.26 270 top
R121  22  [R0402]  33.55,24.26 270 top
R122  22  [R0402]  35.59,24.26 270 top
R123  510  [R0402]  23.42,24.26 270 top
R124  510  [R0402]  24.89,34.16 90 top
R125  22  [R0402]  36.6,24.26 270 top
R126  22  [R0402]  39.65,24.26 270 top
R127  22  [R0402]  38.56,26.85 0 top
R128  1.5K  [R0402]  18.8,3.43 270 top
R129  22  [R0402]  38.56,32.94 0 top
R130  10K  [R0402]  96.49,46.99 90 top
R131  22  [R0402]  38.56,31.93 0 top
R132  22  [R0402]  38.56,30.91 0 top
R133  22  [R0402]  38.56,29.9 0 top
R134  22  [R0402]  38.56,27.86 0 top
R135  22  [R0402]  38.56,28.88 0 top
R136  10K  [R0402]  97.21,33.99 180 top
R137  100K  [R0402]  31.75,12.95 180 top
R138  22  [R0402]  38.56,33.96 0 top
R139  22  [R0402]  38.56,35.99 0 top
R140  27K  [R0402]  95.5,23.39 180 top
R141  10K  [R0402]  27.43,16.76 180 bottom
R142  0, DNI  [R0402]  25.43,24.26 270 top
R143  10K  [R0402]  23.11,16.64 0 bottom
R144  10K  [R0402]  24.41,24.26 270 top
R145  1.5K  [R0402]  38.56,34.98 180 top
R146  100K  [R0402]  33.81,33.71 0 top
R147  1.5K  [R0402]  97.46,46.86 90 bottom
R148  1.5K  [R0402]  98.42,46.86 90 bottom
R149  1K  [R0402]  74.8,22.35 0 top
R150  1K  [R0402]  97.92,13.08 90 top
R151  1K  [R0402]  96.9,13.08 90 top
R152  1K  [R0402]  95.89,13.08 90 top
R153  1K  [R0402]  94.87,13.08 90 top
R154  0, DNI  [R0402]  36.32,16 90 top
R155  100K  [R0402]  45.85,8.26 90 top
R156  0, DNI  [R0402]  36.32,12.95 90 top
R157  1K  [R0402]  39.24,8.26 270 top
R158  100K  [R0402]  40.13,15.75 0 top
R159  0, DNI  [R0402]  48.64,8.89 270 top
R160  10K  [R0402]  44.96,15.75 0 top
R161  10K  [R0402]  37.47,9.4 90 top
R162  0, DNI  [R0402]  48.64,11.94 270 top
R163  1.5K  [R0402]  86.31,26.54 270 bottom
R164  1.5K  [R0402]  85.32,26.57 270 bottom
R165  0  [R0402]  25.91,52.7 90 bottom
R166  50K  [R0402]  27.81,13.72 180 bottom
R167  0  [R0402]  46.48,37.03 180 bottom
R168  DNP  [R0805]  60.96,41.27 90 top
S1  KMR231GLFS  [SW4SMD_63X161LS]  4.45,52.17 0 top
S2  KMR231GLFS  [SW4SMD_63X161LS]  12.06,52.17 0 top
S3  KMR231GLFS  [SW4SMD_63X161LS]  99.57,43.33 0 top
TP1  TPB0,65  [TP_B0,65]  64.14,22.61 0 bottom
TP2  TPB0,65  [TP_B0,65]  64.14,23.62 0 bottom
TP3  TPB0,65  [TP_B0,65]  60.07,22.58 0 bottom
TP4  TPB0,65  [TP_B0,65]  59.05,22.58 0 bottom
TP5  TESTPAD/W_HOLE_1X1  [TESTPAD/W_HOLE_1X1]  31.11,50.16 0 top
TP6  TESTPAD/W_HOLE_1X1  [TESTPAD/W_HOLE_1X1]  28.57,50.16 0 top
TP7  TESTPAD/W_HOLE_1X1  [TESTPAD/W_HOLE_1X1]  31.11,52.7 0 top
TP8  TESTPAD/W_HOLE_1X1  [TESTPAD/W_HOLE_1X1]  28.57,52.7 0 top
TP9  TPB0,65  [TP_B0,65]  24.64,6.73 0 top
TP10  TPB0,65  [TP_B0,65]  28.7,6.73 0 top
TP11  TPB0,65  [TP_B0,65]  63.12,29.13 0 bottom
TP12  TPB0,65  [TP_B0,65]  62.1,22.58 0 bottom
TP13  TPB0,65  [TP_B0,65]  58.04,22.58 0 bottom
TP14  TPB0,65  [TP_B0,65]  52.5,40.06 0 top
TP15  TPB0,65  [TP_B0,65]  58.04,24.13 0 bottom
TP16  TPB0,65  [TP_B0,65]  61.85,24.16 0 bottom
TP17  TPB0,65  [TP_B0,65]  28.85,25.76 0 top
TP18  TESTPAD/W_HOLE_1X1  [TESTPAD/W_HOLE_1X1]  28.57,1.91 0 top
TP19  TESTPAD/W_HOLE_1X1  [TESTPAD/W_HOLE_1X1]  31.11,1.91 0 top
TP20  TESTPAD/W_HOLE_1X1  [TESTPAD/W_HOLE_1X1]  31.11,4.45 0 top
TP21  TPB0,65  [TP_B0,65]  56.87,31.5 0 bottom
TP22  TPB0,65  [TP_B0,65]  65.81,36.83 0 bottom
TP23  TPB0,65  [TP_B0,65]  64.01,28.57 0 bottom
TP24  TPB0,65  [TP_B0,65]  64.16,21.64 0 bottom
TP25  TESTPAD/W_HOLE_1X1  [TESTPAD/W_HOLE_1X1]  34.16,35.81 0 top
TP26  TESTPAD/W_HOLE_1X1  [TESTPAD/W_HOLE_1X1]  53.9,36.68 0 top
TP27  TPB0,65  [TP_B0,65]  46.33,11.81 0 top
TP28  TPB0,65  [TP_B0,65]  46.33,10.54 0 top
TP29  TPB0,65  [TP_B0,65]  38.76,13.08 0 top
TP30  TPB0,65  [TP_B0,65]  38.76,14.35 0 top
U1  OSD3358-512M-BSM  [OSD335X-BGA-256]  60.58,25.15 90 top
U2  TPD4S012DRYR_P1_M  [6-SON(1.45X1)]  10.01,46.56 180 bottom
U3  SN74LVC1G07DCKRG4  [SC-70-5]  54.23,41.53 180 top
U4  BU4240FVE-TR  [5-VSOF(1.6X1.6MM)]  47.98,37.72 0 top
U5  TLVH431NAMQDBZRVL  [SOT23-3]  58.04,28.7 180 bottom
U6  SN74LVC2G241DCUR  [8-VSSOP(2.3X2MM)]  70.18,10.74 0 bottom
U7  THGBMNG5D1LBAIT  [153-WFBGA(11X10)]  73.74,42.34 90 top
U8  USB2534-1080AEN  [6-SQFN(6X6)]  25.65,11.43 0 top
U9  AR8035-AL1A  [40-QFN(5X5MM)]  30.1,29.21 270 top
U10  TDA19988BHN/C1,551  [64-HVQFN(9X9)]  90.3,37.82 0 top
U11  TPD4S012DRYR_P1_P  [6-SON(1.45X1)]  18.41,16.89 0 top
U12  TPD4S012DRYR_P1_P  [6-SON(1.45X1)]  18.41,19.3 0 top
U13  TPD4S012DRYR_P1_P  [6-SON(1.45X1)]  15.62,8.26 270 top
U14  TPD4S012DRYR_P1_P  [6-SON(1.45X1)]  18.03,8.26 270 top
U15  TPS2051BDGN  [8-TSSOP(3.00MM_WIDTH)]  25.4,19.05 0 bottom
U16  AT97SC3205T-G3M4400B  [QFN32-0.4-4X4MM]  82.68,13.97 0 top
U17  TMP468AIYFFR  [16-DSBGA]  92.33,14.73 90 top
U18  SN74LVC2G53YZPR  [8-DSBGA(1.9X0.9)]  37.47,14.86 0 top
U19  SN74LVC2G53YZPR  [8-DSBGA(1.9X0.9)]  37.47,11.81 0 top
U20  SN74LVC2G53YZPR  [8-DSBGA(1.9X0.9)]  47.5,10.03 180 top
U21  S25FL127S  [8-WSON(5X6MM)]  42.55,12.45 0 top
U22  LPS22HBTR  [10-HLGA(2X2MM)]  81.41,25.53 180 top
U23  ICM-20948  [24-QFN(3X3)]  88.52,27.3 0 top
U24  SN74LVC2G53YZPR  [8-DSBGA(1.9X0.9)]  47.5,13.08 180 top
U25  PCA9306DQER  [8-X2SON(1.4X1.0)]  88.9,29.77 180 bottom
U26  TPS22958DGKR  [8-VSSOP(3X3MM)]  47.24,40.26 0 top
U$1  [OCTAVO-LOGO-V2_SM-RED]  40.06,37.54 270 top
U$2  [XYZ-LABEL]  73.79,28.83 0 top
X1  10118192-0001LF  [MICRO_USB_2.0_RECEP_5POS_SMD_RIGHT_ANGLE]  1.45,46.69 90 bottom
X3  DM3BT-DSF-PEJS  [10(8+2)POS_MICRO_SD_SMD_RIGHT_ANGLE]  107.7,19.94 270 bottom
X4  1002-004-01010  [USB_HOST_HORIZONTAL_W/CHASSIS_GND_DUAL]  -3.81,10.54 270 top
X5  RJMG2310228A0ER  [RJ45_10/100/1000_DUAL_USB_A_THRUHOLE_CONN]  -3.81,30.23 270 top
X6  10118241-001RLF  [MICRO_HDMI_19POS_SMD&THRUHOLE_RIGHT_ANGLE]  106.17,39.12 270 bottom
Y1  ABS07-32.768KHZ-T  [2-SMD,NO_LEAD(3.2X1.5MM)]  64.39,11.13 180 top
Y2  7A-24.000MAAJ-T  [2-SMD,NO_LEAD(5X3.2MM)]  46.1,31.5 270 top
Y3  ASDMB-12.000MHZ-LC-T  [4-SMD,NO_LEAD(2.5X2MM)]  92.2,29.08 0 top
Y4  7A-24.000MAAJ-T  [2-SMD,NO_LEAD(5X3.2MM)]  25.4,18.8 0 top
Y5  ASDMB-24.576MHZ-LC-T  [4-SMD,NO_LEAD(2.5X2MM)]  74.9,16.15 90 top
Y6  7A-25.000MAAE-T  [2-SMD,NO_LEAD(5X3.2MM)]  30.38,36.83 180 top

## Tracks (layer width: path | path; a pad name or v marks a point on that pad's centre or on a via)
12MHZ
  Top 0.152: U10.27 91.55,32.89 91.75,32.69 92.53,32.69 92.76,32.46 R102.2
AGND  (via drill 0.3)
  Top 0.152: v58.9,13.03 59.94,14.07 U1.A9
  Bottom 0.152: C8.2 C9.2 55.12,13.41 55.3,13.59 57,13.59 57.15,13.74 C10.2 57.53,14.15 57.66,14.02 57.66,13.18 57.81,13.03 R25.2 v58.9,13.03 58.9,10.59 62.64,6.86 62.64,6.55 63.7,5.49 69.75,5.49 70.26,4.98 70.26,1.32 70.74,0.84 80.01,0.84 80.85,1.68 80.85,2.34 81.92,3.4 J6.34
AIN0  (via drill 0.3)
  Top 0.152: U1.A8 61.21,14.99 61.49,14.71 61.49,12.78 62.05,12.22 62.05,9.96 62.79,9.22 v65.02,9.22 | J6.39 88.47,2.97 88.47,5.31 87.83,5.94 79.1,5.94 v78.64,5.49
  Bottom 0.152: v65.02,9.22 65.56,8.69 67.67,8.69 68.1,8.26 68.1,7.19 68.89,6.4 70.33,6.4 70.94,5.79 75.36,5.79 75.67,6.1 78.03,6.1 v78.64,5.49
AIN1  (via drill 0.3)
  Top 0.152: U1.B8 61.21,16.31 61.8,15.72 61.8,12.9 62.36,12.34 62.36,10.08 62.69,9.75 65.41,9.75 v65.94,9.22 | J6.40 89.53,5.41 88.7,6.25 v78.64,6.25
  Bottom 0.152: v78.64,6.25 78.49,6.4 75.51,6.4 75.21,6.1 71.07,6.1 70.26,6.91 70.26,8.1 69.67,8.69 68.1,8.69 67.56,9.22 v65.94,9.22
AIN2  (via drill 0.3)
  Top 0.152: U1.B6 v63.12,16.26
  Bottom 0.152: v63.12,16.26 64.57,14.81 72.03,14.81 72.62,15.39 74.09,15.39 75.29,14.2 75.29,13.26 79.7,8.84 84.12,8.84 84.58,8.38 84.58,6.4 85.95,5.03 85.95,2.95 J6.37
AIN3  (via drill 0.3)
  Top 0.152: U1.C6 63.35,18.16 63.09,17.91 v63.09,17.3
  Bottom 0.152: v63.09,17.3 65.28,15.11 71.91,15.11 72.49,15.7 74.22,15.7 75.59,14.33 75.59,13.41 79.87,9.13 84.29,9.13 84.89,8.53 84.89,6.55 J6.38
AIN4  (via drill 0.3)
  Top 0.152: U1.C7 62.23,18.16 61.87,17.8 v61.87,17.27
  Bottom 0.152: v61.87,17.27 62.48,16.66 62.48,16.03 64.01,14.5 72.16,14.5 72.75,15.09 73.97,15.09 74.98,14.07 74.98,13.11 79.48,8.61 79.48,6.25 79.78,5.94 82.27,5.94 82.98,5.23 82.98,2.97 J6.33
AIN5  (via drill 0.3)
  Top 0.152: U1.C8 60.73,17.68 60.73,15.04 61.19,14.58 61.19,12.65 61.75,12.09 61.75,9.83 62.89,8.69 67.21,8.69 67.74,8.15 v67.74,6.78 | J6.36 83.26,5.64 80.67,5.64 v80.44,5.41
  Bottom 0.152: v67.74,6.78 68.43,6.1 70.1,6.1 70.71,5.49 72.57,5.49 73.23,4.83 73.23,3.99 73.84,3.38 79.91,3.38 80.44,3.91 v80.44,5.41
AIN6  (via drill 0.3)
  Top 0.152: U1.C9 60.43,17.68 60.43,13.44 v59.44,12.45 | J6.35 83.31,3.05 v80.62,3.05
  Bottom 0.152: v80.62,3.05 71.45,3.05 70.56,3.94 70.56,5.18 69.95,5.79 63.86,5.79 62.94,6.71 62.94,7.01 59.44,10.52 v59.44,12.45
AIN7
  Top 0.152: U1.D6 U1.D7
B_UART0_RX
  Bottom 0.152: J3.4 71.75,8.74 71.55,8.94 70.94,8.94 70.48,9.4 70.48,10.41 71.06,10.99 U6.2 72.32,10.99 72.64,10.67 R27.2
B_UART0_TX
  Bottom 0.152: U6.3 71.05,10.49 70.79,10.24 70.79,9.53 71.07,9.25 73.97,9.25 74.3,8.91 J3.5
BAT_SENSE
  Top 0.152: U1.N7 61.7,31.65 61.7,35.64 62.03,35.97 62.03,43.08 61.52,43.59 52.96,43.59 52.15,44.4 52.15,46.71 51.44,47.42 43.48,47.42 42.98,46.91 42.98,45.14 42.62,44.78 38.71,44.78 38.3,45.19 38.3,46.91 37.41,47.8 33.55,47.8 32.41,48.95 28.8,48.95 28.57,49.17 TP6.P$1
  Bottom 0.152: TP6.P$1 27.13,50.16 25.91,51.38 R165.1
BC_EN1  (via drill 0.3)
  Top 0.152: U8.12 24.65,7.76 v23.62,6.73
  Bottom 0.152: R113.2 v23.62,6.73
BC_EN2  (via drill 0.3)
  Top 0.152: U8.16 26.65,7.76 v27.69,6.73
  Bottom 0.152: R112.2 v27.69,6.73
BC_EN3  (via drill 0.3)
  Top 0.152: U8.18 28.33,8.63 28.7,8.26 v28.7,7.75
  Bottom 0.152: R111.2 v28.7,7.75
BC_EN4
  Top 0.152: U8.20 29.57,9.93 29.97,9.53 29.97,8.38 30.1,8.26 R107.2
CFG_SEL0
  Top 0.152: U8.24 28.9,11.93 28.96,11.99 30.05,11.99 30.61,11.43 30.61,10.92 30.86,10.67 R99.2 31.19,10.19 31.29,10.08 33.3,10.08 33.6,9.78 33.6,7.49 32.92,6.81 31.37,6.81 29.82,5.26 26.85,5.26 J8.2
CFG_SEL1
  Top 0.152: TP20.P$1 31.11,5.84 31.77,6.5 33.05,6.5 33.91,7.37 33.91,10.79 33.48,11.23 31.29,11.23 31.19,11.33 R97.2 30.73,11.81 30.11,12.43 U8.25
CGND
  Bottom 0.152: X3.CGND3 107.45,26.19 X3.CGND1
  Bottom 0.813: X3.CGND4 91.77,25.02 92.71,25.02 93.22,24.51 93.22,23.62 96.27,20.57 106.93,20.57 | X3.CGND5 95.95,14.54 96.39,14.99 106.17,14.99
  pour Top: 6.99,27.3 -5.08,27.3 -5.08,-5.08 113.03,-5.08 113.03,27.3 106.68,27.3 106.68,10.16 106.05,9.53 100.97,9.53 99.06,7.62 99.06,0.64 40.01,0.64 39.37,1.27 39.37,5.08 38.1,6.35 34.29,6.35 33.02,5.08 33.02,1.27 32.38,0.64 15.24,0.64 14.61,1.27 14.61,3.81 13.97,4.45 6.99,4.45 6.99,16.51 13.97,16.51 14.61,17.14 14.61,19.18 16.51,21.08 16.51,23.5 15.88,24.13 6.99,24.13
  pour Bottom (rank 6): -1.27,27.3 6.73,27.3 6.73,42.8 5.08,44.45 3.05,44.45 3.05,48.9 5.08,48.9 6.35,50.16 6.35,53.98 32.38,53.98 33.02,53.34 33.02,49.53 34.29,48.26 38.1,48.26 39.37,49.53 39.37,53.34 40.01,53.98 98.42,53.98 99.06,53.34 99.06,46.99 100.97,45.09 101.6,45.09 102.23,44.45 102.23,41.27 104.14,41.27 104.78,40.64 106.68,40.64 106.68,37.47 104.78,37.47 104.14,36.83 102.23,36.83 102.23,34.29 103.5,33.15 106.05,33.15 106.68,32.51 106.68,29.21 106.05,28.57 106.05,27.3 109.22,27.3 109.22,55.88 -1.27,55.88
  pour Bottom (rank 6): 6.73,27.3 -1.27,27.3 -1.27,-1.27 109.22,-1.27 109.22,27.3 106.05,27.3 106.05,15.75 105.54,15.24 103.76,15.24 103.12,14.61 103.12,12.83 103.76,12.19 105.66,12.19 106.05,11.81 106.05,10.16 105.41,9.53 100.97,9.53 99.06,7.62 99.06,1.27 98.42,0.64 40.01,0.64 39.37,1.27 39.37,5.08 38.1,6.35 34.29,6.35 33.02,5.08 33.02,1.27 32.38,0.64 7.62,0.64 6.73,1.52
  pour Top: -5.08,27.3 6.99,27.3 6.99,36.2 15.24,36.2 16.51,37.47 16.51,38.73 15.24,40.01 1.91,40.01 1.27,40.64 1.27,53.34 1.91,53.98 14.48,53.98 14.99,53.47 14.99,50.8 14.73,50.55 13.46,50.55 13.21,50.29 13.21,49.28 15.88,49.28 16.51,49.91 16.51,53.47 17.02,53.98 32.38,53.98 33.02,53.34 33.02,49.53 34.29,48.26 38.1,48.26 39.37,49.53 39.37,53.34 40.01,53.98 99.06,53.98 99.06,46.99 100.97,45.09 103.5,45.09 104.14,44.45 104.14,41.27 104.78,40.64 106.68,40.64 106.68,37.47 104.78,37.47 104.14,36.83 104.14,35.05 106.68,32.51 106.68,27.3 113.03,27.3 113.03,59.69 -5.08,59.69
CLK_25M
  Top 0.152: U9.23 29.1,26 TP17.TP
CLKOUT2  (via drill 0.3)
  Top 0.152: C2.2 68.62,12.15 68.45,12.32 R3.2 R7.2 69.52,12.7 70.03,12.7 v70.21,12.88 | v73.69,13.64 v76.2,13.64 | J6.41 93.14,2.97 98.02,2.97 98.75,3.71 98.75,7.72 100.79,9.75 105.92,9.75 106.48,10.31 106.48,31.01 105.74,31.75 102.36,31.75 101.73,31.11 J4.18
  Bottom 0.152: v70.21,12.88 72.24,12.88 73,13.64 v73.69,13.64 | v76.2,13.64 76.78,13.64 77.27,14.12 80.82,14.12 84.28,10.67 84.28,9.6 85.19,8.69 85.19,6.71 86.41,5.49 90.35,5.49 90.98,4.85 90.98,3 J6.41
DCAN1_RX/TPM_GPIO2  (via drill 0.3)
  Top 0.152: v73.69,12.47 74.4,12.47 74.68,12.75 76.56,12.75 78,14.2 80.16,14.2 80.19,14.17 U16.4 | U1.C13 55.65,17.37 57.61,17.37 57.89,17.09 57.89,14.88 56.54,13.54 56.54,10.52 57.15,9.91 59.35,9.91 60.29,10.85 v60.81,10.85 60.81,9.98 60.12,9.3 57.15,9.3 56.52,8.66 J12.1
  Bottom 0.152: v73.69,12.47 72.69,12.47 72.26,12.04 67.11,12.04 65.91,10.85 v60.81,10.85
DCAN1_TX/TPM_GPIO1  (via drill 0.3)
  Top 0.152: U1.C12 56.13,17.91 56.36,17.68 57.73,17.68 58.19,17.22 58.19,14.76 56.84,13.41 56.84,10.62 57.25,10.21 59.26,10.21 60.6,11.56 v61.21,11.56 61.42,11.35 61.42,9.98 J12.2 | v73.18,13.06 76.43,13.06 77.88,14.5 80.19,14.5 80.25,14.57 U16.3
  Bottom 0.152: v73.18,13.06 72.85,13.06 72.14,12.34 66.98,12.34 66.19,11.56 v61.21,11.56
DVI_+5V  (via drill 0.3)
  Top 0.254: v101.17,41.48 101.02,41.63 100.51,41.63 100.23,41.91 v100.23,44.09 v99.16,44.09
  Bottom 0.152: R148.2 R147.2
  Bottom 0.254: R148.2 98.98,47.42 99.26,47.14 99.26,45.77 100.23,44.81 v100.23,44.09 | X6.10 101.4,41.25 v101.17,41.48
  other vias: 79.91,30.81 79.91,29.74
  pour Bottom (no thermals): 78.03,29.31 78.03,31.22 80.31,31.22 80.31,29.31
  pour Route15: 100.61,44.48 100.61,43.71 96.9,43.71 96.16,42.98 93.12,42.98 92.02,44.07 84.86,44.07 83.72,42.93 83.72,33.32 82.47,32.08 80.59,32.08 80.31,31.8 80.31,29.31 79.5,29.31 79.5,32.21 80.39,33.1 81.86,33.1 82.8,34.04 82.8,43.1 84.66,44.96 92.23,44.96 93.62,43.56 95.76,43.56 96.67,44.48
  pour Bottom (no thermals): 100.94,40.79 101.83,40.79 101.83,41.76 100.94,41.76
  pour Top (no thermals): 98.96,43.64 99.77,43.64 99.9,43.51 99.9,41.78 100.61,41.07 101.45,41.07 101.45,41.78 100.41,41.78 100.25,41.94 100.25,43.59 100.48,43.81 100.48,44.35 98.96,44.35
EEPROM_WP  (via drill 0.3)
  Top 0.152: U1.M2 68.43,29.18 v68.25,29.18
  Bottom 0.152: v68.25,29.18 67.59,29.18 65.53,31.24 65.53,32.16 62.33,35.36 62.33,41.33 60.53,43.13 52.45,43.13 50.9,44.68 50.9,45.95 50.49,46.35 J1.1
EHRPWM1A  (via drill 0.3)
  Top 0.152: U1.P12 v55.37,32.89
  Bottom 0.152: J6.14 56.52,5.38 56.29,5.61 53.44,5.61 52.22,6.83 52.22,12.62 49.76,15.09 49.76,22.5 51.79,24.54 51.79,30 52.63,30.84 52.98,30.84 55.04,32.89 v55.37,32.89
EHRPWM1B  (via drill 0.3)
  Top 0.152: U1.T13 54.86,34.27 55.14,33.98 v55.37,33.98
  Bottom 0.152: J6.16 59.05,5.49 58.6,5.94 53.54,5.94 52.53,6.96 52.53,12.75 50.06,15.21 50.06,22.38 52.09,24.41 52.09,29.87 52.76,30.53 53.11,30.53 54.89,32.31 55.65,32.31 55.93,32.59 55.93,33.6 55.55,33.98 v55.37,33.98
EHRPWM2A
  Top 0.152: J5.19 64.14,47.04 65.08,46.1 65.08,37.49 66.47,36.09 66.47,35.53 66.29,35.36 U1.T4
EHRPWM2B  (via drill 0.3)
  Top 0.152: U1.P5 64.54,32.61 64.54,35.46 64.16,35.84 64.16,45.72 61.72,48.16 v61.11,48.16
  Bottom 0.152: J5.13 56.52,48.79 57.15,48.16 v61.11,48.16
EMMC_RSTN  (via drill 0.3)
  Top 0.127: 74.99,40.75 U7.K5
  Top 0.152: v74.47,38.43 74.47,39.08 U7.J1 U7.J2 U7.J3 74.49,40.25 74.99,40.75
  Bottom 0.152: R52.1 R19.2 74.68,37.54 74.47,37.74 v74.47,38.43
EMMC_VCCI  (via drill 0.3)
  Top 0.152: v71.48,38.43 arc90 71.49,38.44 U7.C1 U7.C2
  Bottom 0.152: C13.2 71.48,38.18 v71.48,38.43
ETH_AVDDL  (via drill 0.3)
  Top 0.152: v29.74,32.56 29.9,32.41 U9.6
  Top 0.203: U9.11 27.7,31.23 27.41,31.52 v27.2,31.52 | U9.17 26.73,28.61 v26.57,28.45
  Bottom 0.203: C66.1 27.1,31.42 v27.2,31.52 27.1,31.62 C67.1 | FB2.1 C68.1 26.04,27.91 v26.57,28.45
  pour Route15 (no thermals): 26.06,28.85 26.06,28.27 29.49,28.27 29.69,28.47 29.69,30.84 29.95,31.09 29.95,33.05 29.39,33.05 29.39,31.75 29.16,31.52 28.04,31.52 27.76,31.8 26.87,31.8 26.87,31.14 28.14,31.14 28.14,28.85
ETH_DVDDL  (via drill 0.3)
  Top 0.203: U9.38 35.44,30.21 v35.56,30.33
  Bottom 0.152: L1.P$2 31.75,30.97 31.98,30.73 32.33,30.73 32.64,30.43 C72.1
  Bottom 0.203: FB2.2 27.81,25.76 28.19,25.38 31.37,25.38 31.77,25.78 31.77,29.39 31.98,29.59 C72.1 33.3,29.59 33.5,29.79 33.5,30.56 33.71,30.76 35.13,30.76 v35.56,30.33
  Bottom 0.305: C70.1 v35.56,30.33 36.27,30.33 36.58,30.02 C71.1
ETH_INT
  Top 0.152: R144.1 R142.1 25.43,25.68 27.16,27.41 U9.20
ETH_LX  (via drill 0.3)
  Top 0.152: U9.2 31.5,32.03 31.62,32.16 v33.02,32.16
  Bottom 0.152: v33.02,32.16 33.2,32.16 33.35,32 L1.P$1
ETH_VDDIO  (via drill 0.3)
  Top 0.152: U9.8 29.1,31.94 28.85,32.18 28.85,32.51 v28.68,32.69 28.3,32.69 27.38,33.6 26.64,33.6 26.52,33.48 26.52,33.12 26.39,32.99 25.6,32.99 25.45,33.15 25.45,35.71 R104.1
  Top 0.203: U9.27 30.7,25.98 v30.66,25.93
  Bottom 0.152: C65.1 29.52,31.85 v28.68,32.69 29.13,33.15 29.34,33.15 29.52,33.33 C64.1
  Bottom 0.203: C65.1 30.24,31.3 30.66,30.89 v30.66,25.93
FLASH_EN  (via drill 0.3)
  Top 0.152: U1.J14 53.29,25.48 v53.29,25.2 | U18.D2 38.11,13.72 40.31,13.72 40.56,13.46 40.56,12.62 | U19.D2 39.1,12.45 40.39,12.45 | 40.39,12.45 40.56,12.45 | 40.56,12.62 40.56,12.45 | 40.56,12.45 40.56,12.27 | 40.56,12.27 40.56,10.77 40.74,10.59 42.82,10.59 43.79,9.63 | 43.81,9.6 J11.2 45.77,7.62 R155.1 53.44,7.7 v53.67,7.47 | U20.D2 46.85,11.18 44.76,11.18 | 44.76,11.18 44.53,11.18 | 44.53,11.4 44.53,12.19 44.78,12.45 45.86,12.45 U24.D2 | 44.53,11.4 44.53,11.18 | 44.53,11.18 44.53,10.95 | 44.53,10.95 44.53,10.31 43.81,9.6 | 40.39,12.45 40.56,12.62 | 40.39,12.45 40.56,12.27 | 44.76,11.18 44.53,11.4 | 44.76,11.18 44.53,10.95 | 43.69,9.75 43.79,9.75 | 43.79,9.75 43.94,9.75 | 43.81,9.6 43.79,9.63 | 43.79,9.63 43.79,9.75
  Bottom 0.152: v53.29,25.2 53.29,25.04 53.01,24.77 53.01,24.03 50.98,22 50.98,15.6 53.44,13.13 53.44,7.7 v53.67,7.47
GND  (via drill 0.3, 0.3 pad 0.61, 0.5)
  Top 0.127: U7.N5 U7.P4 | 72.97,39.09 U7.C4 | U7.D3 U7.E2 U7.F1 72.97,39.08 72.97,38.91
  Top 0.152: C48.2 v16.89,11.43 | R128.1 v18.8,4.83 | C73.2 v15.85,4.65 | R105.1 v33.07,14.1 | R103.1 v33.07,9.53 | R99.1 v33.07,10.67 | R97.1 v33.07,11.81 | R106.1 v34.57,22.94 | R101.2 v38.63,22.94 | U17.B4 U17.A4 91.73,13.75 91.54,13.56 v91.19,13.56 | U16.9 81.11,12.07 80.82,11.79 v80.82,11.61 | U16.24 85.04,15.37 v85.22,15.19 85,14.97 U16.23 | U16.18 85.03,12.97 v85.22,13.16 85,13.37 U16.19 | U16.20 85.02,13.77 v85.22,13.97 85.02,14.17 U16.21 | C85.2 v86.72,12.5 | C86.2 v93.98,12.45 | U16.2 80.18,14.97 v80.03,15.11 | U16.5 80.27,13.77 v80.06,13.56 80.25,13.37 U16.6 | R118.1 v97.46,48.36 | C15.2 101.65,33.98 101.96,33.68 v101.96,33.38 | R136.1 98.27,33.98 98.73,33.53 v98.73,33.4 | S3.4 98.26,42.53 v98.45,42.72 | U7.P6 77.31,41.59 v77.6,41.3 | C45.2 v28.47,22.94 | R109.1 v37.62,22.94 | C44.2 v26.44,22.94 | S1.2 7.46,51.37 v7.47,51.38 | S2.3 8.95,52.97 v8.94,52.96 | S3.2 101,42.53 100.81,42.72 v100.81,43.33 | U16.32 81.28,16.18 81.03,16.43 v80.75,16.43 | Y5.2 76.42,16.98 v76.58,17.14 76.58,16.38 76.71,16.26 C87.2 | v30.33,7.72 31.55,7.72 31.75,7.92 31.75,8.15 31.85,8.26 R107.1 | U18.B1 U18.C1 U18.D1 37.07,14.11 v36.58,14.61 37.08,15.11 U18.B1 | R155.2 45.85,9.53 46.05,9.73 v46.38,9.73 | v77.88,39.78 77.06,40.59 U7.P4 | v72.72,37.85 72.97,38.1 72.97,38.91 72.97,39.09 | U23.18 90.09,28.38 v90.09,28.91 90.09,29.21 89.94,29.36 89.18,29.36 89.13,29.31 89.13,28.82 U23.20 | U23.9 88.32,24.84 v88.06,24.59 | C94.2 55.3,39.8 55.45,39.65 v55.45,39.04 | U3.3 56.63,42.18 57.02,41.78 v57.02,41.02 | U7.N2 U7.N1 | U19.C1 U19.D1 37.07,11.06 v36.58,11.56 37.08,12.06 U19.B1 U19.C1 | v48.39,10.29 47.89,10.78 U20.D1 U20.C1 U20.B1 47.88,9.78 v48.39,10.29
  Top 0.152: v48.39,13.34 47.89,13.83 U24.D1 U24.C1 U24.B1 47.88,12.83 v48.39,13.34
  Top 0.203: C60.2 34.06,34.72 v34.37,34.42 | v83.62,32.82 85.83,32.82 | v27.1,35.43 27.51,35.03 C47.2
